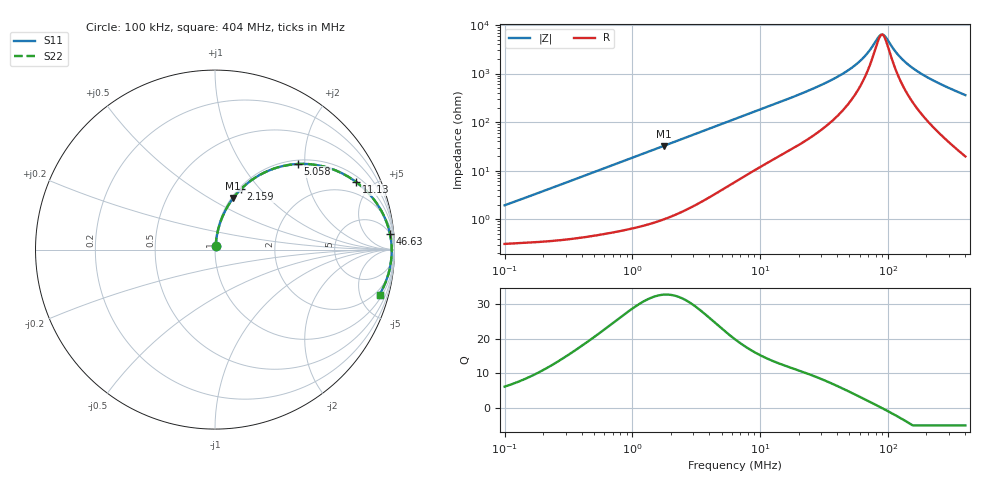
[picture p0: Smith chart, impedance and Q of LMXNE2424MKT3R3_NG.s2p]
! LMXNE2424MKT3R3_NG  S-PARAMETER MODEL  ( General Type )
! Model Generated by TAIYO YUDEN Corporation (https://www.yuden.co.jp/en/)
! Version 1.0
! TAIYO YUDEN Control No. 191023NI43SB-FBB
! Copyright(c) 2019 TAIYO YUDEN CO.,LTD. All Rights Reserved.
! Product Description (link to TY-COMPAS)
! https://ds.yuden.co.jp/TYCOMPAS/or/detail?pn=LMXNE2424MKT3R3MNG&u=M
! Products Name : Inductors
! Characteristics :
!  Inductance : 3.3 uH , SRF(min) : 56 MHz , DC Resistance(max) : 0.27 Ohm
!  Rated Current : Saturation :1400 mA , Temp Rise : 750 mA (40 degC)
!  Case Size : 2.4 x 2.4 / 0.095 x 0.095 [mm/inch] , Thickness : 1.2 / 0.047 [mm/inch]
!  (Conditions: Temperature = 25 degC , DC Bias Current/Voltage = 0A / 0V)
! External Node Assignments :
!  1  o---GGG---o  2
! GND o---------o GND
! Frequency Range : 0.1MHz  -  403.964729MHz  [ 402 STEP ]
# MHz S RI R 50
! Freq[MHz].  S11 Real  S11 Imag  S21 Real  S21 Imag  S12 Real  S12 Imag  S22 Real  S22 Imag
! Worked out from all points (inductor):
!   401 points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, 100 kHz to 404 MHz, reference 50 ohm
!   read as one part in series: L = 3.03 uH near 104.2 kHz
!   highest Q = 32.6 at 1.755 MHz (marker M1), where L = 2.93 uH
!   self-resonance near 88.75 MHz
!   S11 on the Smith chart (normalised r, x): 100 kHz: 1.01, +0.04; 2.159 MHz: 1.02, +0.79; 5.058 MHz: 1.08, +1.85; 11.13 MHz: 1.28, +4.02; 46.63 MHz: 5, +21; 404 MHz: 1.39, -7.19
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0.1  0.00346 0.019  0.9965 -0.019  0.9965 -0.019  0.00346 0.019
0.401849  0.00972 0.0741  0.9903 -0.0741  0.9903 -0.0741  0.00972 0.0741
0.831032  0.0285 0.1487  0.9715 -0.1487  0.9715 -0.1487  0.0285 0.1487
1.614823  0.0883 0.2687  0.9117 -0.2687  0.9117 -0.2687  0.0883 0.2687
1.754642  0.1017 0.2874  0.8983 -0.2874  0.8983 -0.2874  0.1017 0.2874
2.15947  0.1439 0.3359  0.8561 -0.3359  0.8561 -0.3359  0.1439 0.3359
3.203675  0.2641 0.4239  0.7359 -0.4239  0.7359 -0.4239  0.2641 0.4239
5.058215  0.4627 0.4771  0.5373 -0.4771  0.5373 -0.4771  0.4627 0.4771
6.355822  0.5698 0.4705  0.4302 -0.4705  0.4302 -0.4705  0.5698 0.4705
11.13269  0.7868 0.3762  0.2132 -0.3762  0.2132 -0.3762  0.7868 0.3762
16.51586  0.881 0.2844  0.119 -0.2844  0.119 -0.2844  0.881 0.2844
25.54079  0.94 0.1903  0.06 -0.1903  0.06 -0.1903  0.94 0.1903
46.63309  0.9751 0.0872  0.0249 -0.0872  0.0249 -0.0872  0.9751 0.0872
56.21301  0.9798 0.0607  0.0202 -0.0607  0.0202 -0.0607  0.9798 0.0607
65.00517  0.9823 0.0413  0.0177 -0.0413  0.0177 -0.0413  0.9823 0.0413
86.93005  0.9845 0.00424  0.0155 -0.00424  0.0155 -0.00424  0.9845 0.00424
92.51614  0.9846 -0.00359  0.0154 0.00359  0.0154 0.00359  0.9846 -0.00359
102.6353  0.9845 -0.0167  0.0155 0.0167  0.0155 0.0167  0.9845 -0.0167
126.3151  0.983 -0.0436  0.017 0.0436  0.017 0.0436  0.983 -0.0436
165.448  0.9783 -0.0811  0.0217 0.0811  0.0217 0.0811  0.9783 -0.0811
245.4499  0.9631 -0.1457  0.0369 0.1457  0.0369 0.1457  0.9631 -0.1457
403.9647  0.9166 -0.2505  0.0834 0.2505  0.0834 0.2505  0.9166 -0.2505
